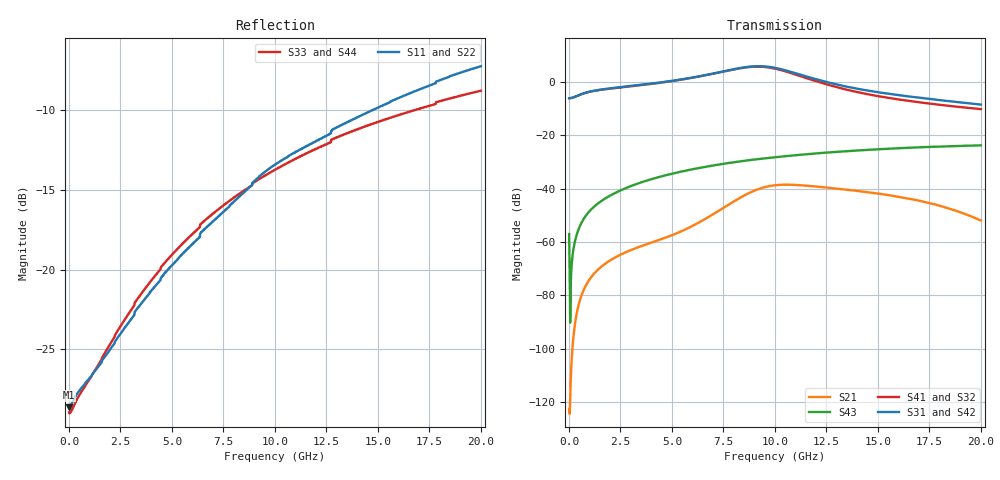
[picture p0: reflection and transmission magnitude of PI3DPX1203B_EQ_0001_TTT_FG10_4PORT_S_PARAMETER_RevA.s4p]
! NPort=4 DATA=2000 NOISE=0 GROUPDELAY=0 COMPLEX_DATAFORMAT=POLAR
! NumOfBlock=1 NumOfParam=0
! .MODEL Smodel S TSTONEFILE=PI3DPX1203B_EQ_0001_TTT_FG10_4PORT_S_PARAMETER_RevA.s4p TYPE=S
!  -- The above .MODEL line can be used for the S element in the netlist.
! The s parameter is extracted from the linear redriver, it is not bi-directional; only s(4,1)s(4,2) and s(3,1)s(3,2)
! should be the insertion loss
!Port definition:
!Port1 = input+
!Port2 = input-
!Port3 = output+
!Port4 = output-
# Hz S MA R  50
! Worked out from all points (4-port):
!   2000 points, 10 MHz to 20 GHz, reference 50 ohm
!   strongest paths, dB at 10 MHz, 5.01 GHz, 10.01 GHz, 15.01 GHz, 20 GHz:
!     S31: -6.2, 0.3, 5.2, -3.9, -8.6
!     S42: -6.2, 0.3, 5.2, -3.9, -8.5
!     S41: -6.2, 0.2, 4.9, -5.4, -10.3
!     S32: -6.2, 0.2, 4.9, -5.4, -10.2
!     S43: -57.1, -34.4, -28.3, -25.3, -23.8
!     S21: -122.7, -57.4, -38.8, -41.9, -52.0
!   lowest |S11| = -28.6 dB at 10 MHz (marker M1), VSWR 1.08, Z = 46.4 - j0.0306 ohm
!   |S11| at or under -10 dB: start of sweep to 14.74 GHz
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1e7  0.03701 -179.5  7.338e-07 10.5  0 0.0  0 0.0
     7.338e-07 10.5  0.03701 -179.5  0 0.0  0 0.0
     0.4917 -0.2  0.4917 179.8  0.03566 178.2  0.001403 -77.8
     0.4917 179.8  0.4917 -0.2  0.001403 -77.8  0.03566 178.2
1.58e9  0.05109 -144.6  0.0003457 112.9  5.34e-12 75.0  5.085e-11 115.5
        0.0003457 112.9  0.05109 -144.6  5.085e-11 115.5  5.34e-12 75.0
        0.7143 -0.6  0.7077 179.3  0.05212 -142.0  0.005859 82.8
        0.7077 179.3  0.7143 -0.6  0.005859 82.8  0.05212 -142.0
6.18e9  0.1235 -111.4  0.002172 122.8  1.62e-08 -108.1  1.563e-07 66.7
        0.002171 122.8  0.1235 -111.4  1.562e-07 66.7  1.621e-08 -108.1
        1.232 -50.8  1.224 131.8  0.1325 -116.9  0.02371 64.3
        1.224 131.8  1.231 -50.8  0.02371 64.3  0.1325 -116.9
8.68e9  0.1791 -106.4  0.008007 100.5  4.343e-07 160.6  1.232e-06 16.5
        0.008002 100.5  0.1791 -106.4  1.23e-06 16.5  4.344e-07 160.7
        1.897 -102.5  1.868 79.7  0.1802 -115.9  0.03367 51.4
        1.869 79.7  1.896 -102.6  0.03367 51.4  0.1802 -115.9
1.013e10  0.2158 -107.4  0.01164 58.9  1.364e-06 97.6  2.404e-06 -21.6
          0.01163 59.0  0.2158 -107.4  2.4e-06 -21.5  1.364e-06 97.6
          1.777 -148.8  1.71 33.2  0.2077 -116.3  0.03895 43.7
          1.712 33.2  1.776 -148.8  0.03895 43.7  0.2077 -116.3
1.223e10  0.2572 -108.6  0.01069 14.9  3.2e-06 31.6  4.218e-06 -49.8
          0.01068 15.0  0.2572 -108.6  4.218e-06 -49.6  3.202e-06 31.7
          1.054 168.1  0.9591 -9.0  0.2426 -117.6  0.04619 33.0
          0.9605 -9.1  1.053 168.2  0.04619 33.0  0.2426 -117.6
2e10  0.4343 -116.3  0.002521 -45.1  2.175e-05 -105.7  3.281e-05 -134.1
      0.002524 -44.4  0.4344 -116.3  3.29e-05 -134.1  2.178e-05 -105.7
      0.373 87.8  0.3073 -71.6  0.3637 -123.9  0.06431 -7.1
      0.3067 -71.8  0.3738 87.8  0.06431 -7.1  0.3637 -123.9
